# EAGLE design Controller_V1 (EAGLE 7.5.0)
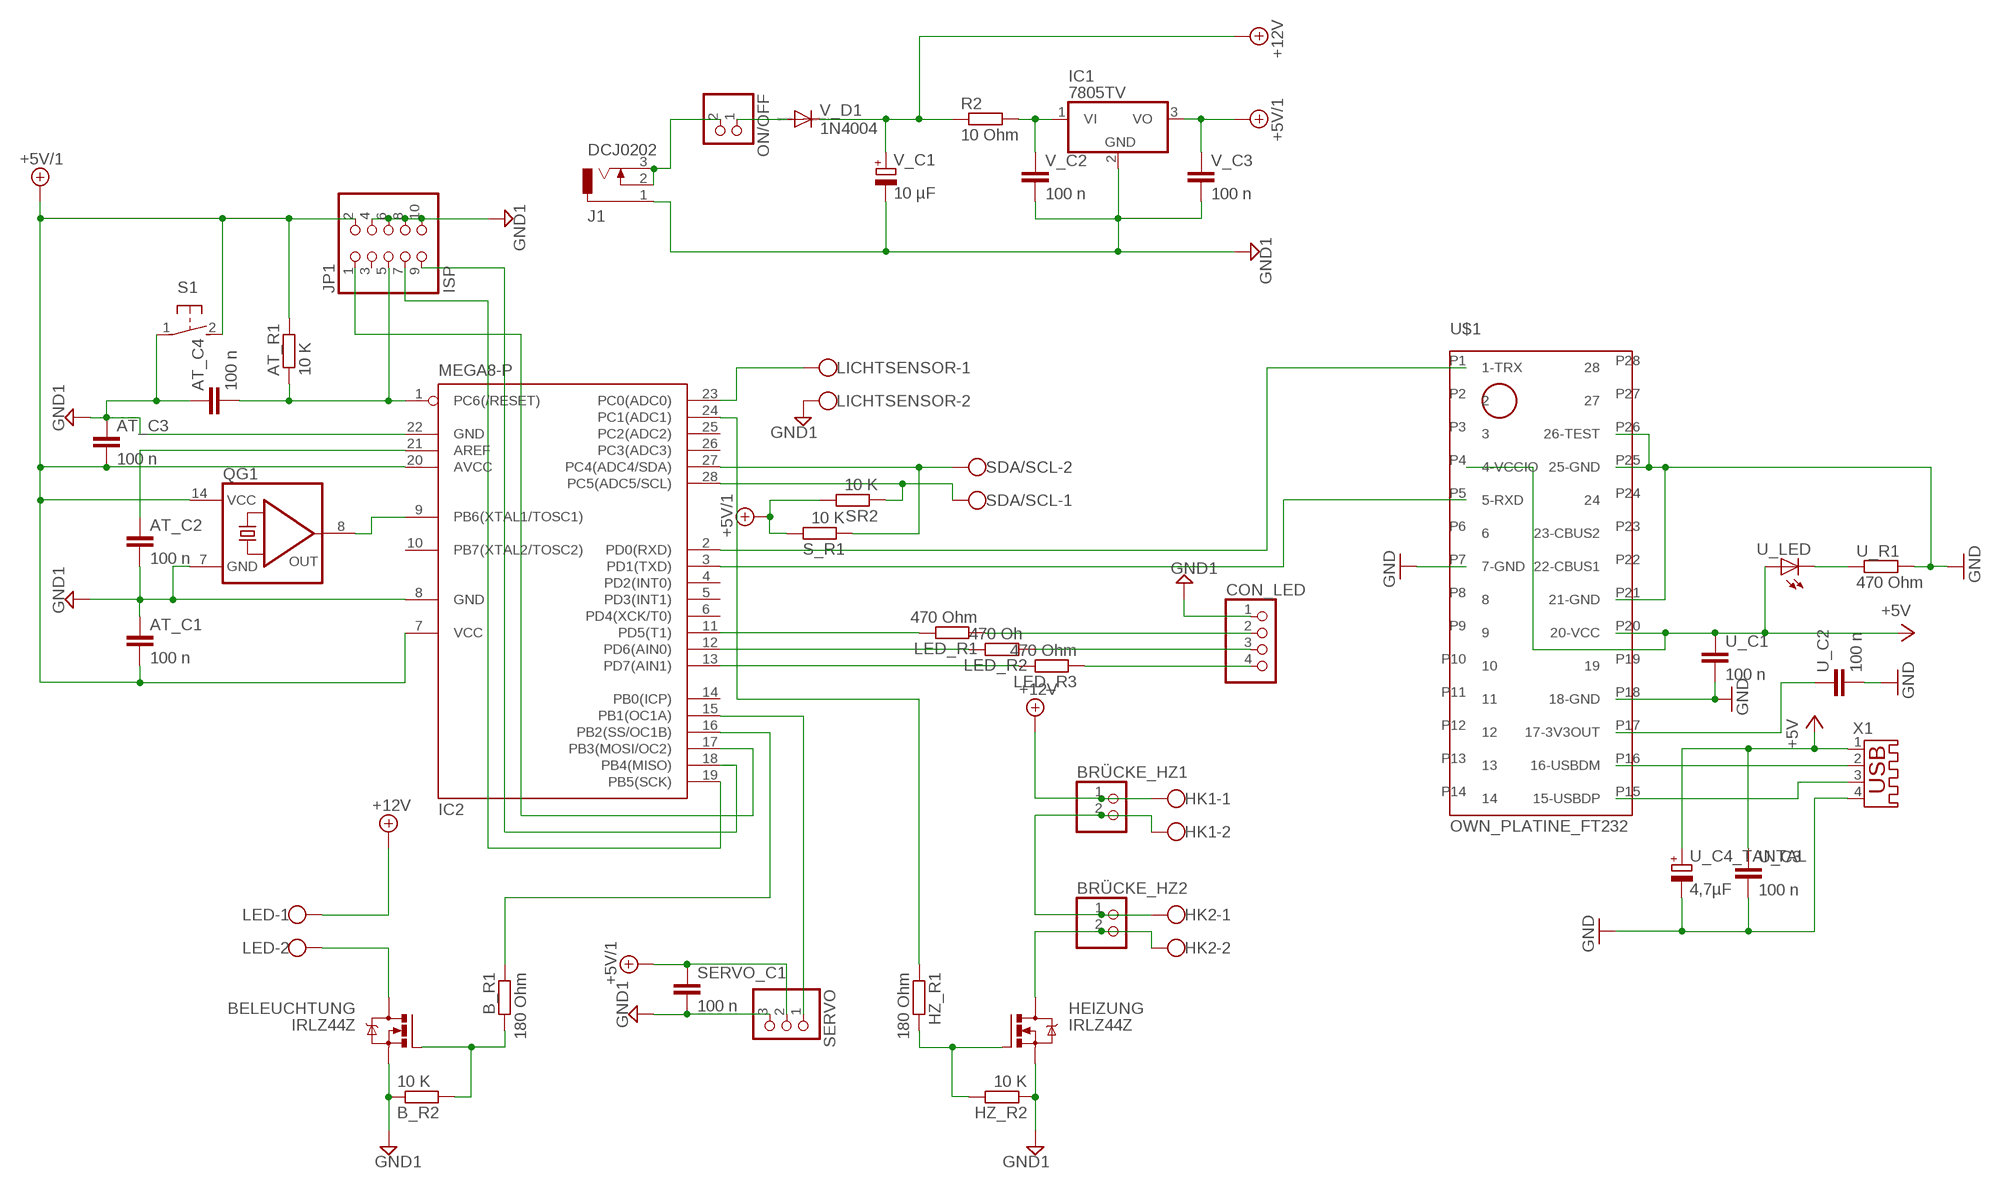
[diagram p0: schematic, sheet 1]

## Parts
AT_C1  100 n  C-EU025-025X050  [C025-025X050]
AT_C2  100 n  C-EU025-025X050  [C025-025X050]
AT_C3  100 n  C-EU025-025X050  [C025-025X050]
AT_C4  100 n  C-EU025-025X050  [C025-025X050]
AT_R1  10 K  R-EU_0204/7  [0204/7]
B_R1  180 Ohm  R-EU_0204/7  [0204/7]
B_R2  10 K  R-EU_0204/7  [0204/7]
BELEUCHTUNG  IRLZ44Z  [TO220BH]
BRÜCKE_HZ1  PINHD-1X2  [1X02]
BRÜCKE_HZ2  PINHD-1X2  [1X02]
CON_LED  PINHD-1X4  [1X04]
HEIZUNG  IRLZ44Z  [TO220BH]
HK1  W237-102  [W237-102]
HK2  W237-102  [W237-102]
HZ_R1  180 Ohm  R-EU_0204/7  [0204/7]
HZ_R2  10 K  R-EU_0204/7  [0204/7]
IC1  7805TV  [TO220V]
IC2  MEGA8-P  [DIL28-3]
J1  DCJ0202  [DCJ0202]
JP1  ISP  PINHD-2X5  [2X05]
LED  W237-102  [W237-102]
LED_R1  470 Ohm  R-EU_0204/7  [0204/7]
LED_R2  470 Oh  R-EU_0204/7  [0204/7]
LED_R3  470 Ohm  R-EU_0204/7  [0204/7]
LICHTSENSOR  W237-102  [W237-102]
ON/OFF  PINHD-1X2  [1X02]
QG1  QG5860  [DIL14S]
R2  10 Ohm  R-EU_0204/7  [0204/7]
S1  31-XX  [B3F-31XX]
S_R1  10 K  R-EU_0204/7  [0204/7]
SDA/SCL  W237-102  [W237-102]
SERVO  PINHD-1X3  [1X03]
SERVO_C1  100 n  C-EU025-025X050  [C025-025X050]
SR2  10 K  R-EU_0204/7  [0204/7]
U$1  OWN_PLATINE_FT232  [OWN_PLATINE_FT232]
U_C1  100 n  C-EU025-025X050  [C025-025X050]
U_C2  100 n  C-EU025-025X050  [C025-025X050]
U_C3  100 n  C-EU025-025X050  [C025-025X050]
U_C4_TANTAL  4,7µF  CPOL-EUE2,5-6E  [E2,5-6E]
U_LED  LED3MM  [LED3MM]
U_R1  470 Ohm  R-EU_0204/7  [0204/7]
V_C1  10 µF  CPOL-EUE2,5-6E  [E2,5-6E]
V_C2  100 n  C-EU025-025X050  [C025-025X050]
V_C3  100 n  C-EU025-025X050  [C025-025X050]
V_D1  1N4004  [DO41-10]
X1  USB-A003  [USB-A003]

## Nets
+5V: U$1.P4(4-VCCIO) U$1.P20(20-VCC) U_C1.1 U_C3.1 U_C4_TANTAL.+ U_LED.A X1.1
+5V/1: AT_C1.2 AT_C3.2 AT_R1.2 IC1.3(VO) IC2.7(VCC) IC2.20(AVCC) JP1.2 QG1.14(VCC) S1.2(S) S_R1.2 SERVO.2 SERVO_C1.1 SR2.2 V_C3.1
+12V: BRÜCKE_HZ1.1 HK1.1 LED.1 R2.1 V_C1.+ V_D1.C
AT_C1: IC2.2(PD0(RXD)) U$1.P1(1-TRX)
BELEUCHTUNG: BELEUCHTUNG.D LED.2
GND: U$1.P7(7-GND) U$1.P18(18-GND) U$1.P21(21-GND) U$1.P25(25-GND) U$1.P26(26-TEST) U_C1.2 U_C2.2 U_C3.2 U_C4_TANTAL.- U_R1.2 X1.4
GND1: AT_C1.1 AT_C2.2 AT_C3.1 AT_C4.1 B_R2.1 BELEUCHTUNG.S CON_LED.1 HEIZUNG.S HZ_R2.1 IC1.2(GND) IC2.8(GND) IC2.22(GND) J1.1 JP1.4 JP1.6 JP1.8 JP1.10 LICHTSENSOR.2 QG1.7(GND) S1.1(P) SERVO.3 SERVO_C1.2 V_C1.- V_C2.2 V_C3.2
N$1: U$1.P15(15-USBDP) X1.3
N$2: U$1.P17(17-3V3OUT) U_C2.1
N$3: U$1.P16(16-USBDM) X1.2
N$4: U_LED.K(C) U_R1.1
N$5: IC2.9(PB6(XTAL1/TOSC1)) QG1.8(OUT)
N$6: AT_C4.2 AT_R1.1 IC2.1(PC6(/RESET)) JP1.5
N$7: IC1.1(VI) R2.2 V_C2.1
N$9: AT_C2.1 IC2.21(AREF)
N$10: IC2.18(PB4(MISO)) JP1.9
N$11: J1.2 J1.3 ON/OFF.2
N$12: IC2.17(PB3(MOSI/OC2)) JP1.1
N$13: IC2.19(PB5(SCK)) JP1.7
N$14: IC2.3(PD1(TXD)) U$1.P5(5-RXD)
N$15: IC2.27(PC4(ADC4/SDA)) S_R1.1 SDA/SCL.2
N$16: IC2.28(PC5(ADC5/SCL)) SDA/SCL.1 SR2.1
N$17: IC2.15(PB1(OC1A)) SERVO.1
N$18: BRÜCKE_HZ1.2 BRÜCKE_HZ2.1 HK1.2 HK2.1
N$19: B_R1.2 B_R2.2 BELEUCHTUNG.G
N$20: HEIZUNG.G HZ_R1.2 HZ_R2.2
N$21: B_R1.1 IC2.16(PB2(SS/OC1B))
N$22: IC2.23(PC0(ADC0)) LICHTSENSOR.1
N$23: HZ_R1.1 IC2.24(PC1(ADC1))
N$24: BRÜCKE_HZ2.2 HEIZUNG.D HK2.2
N$25: IC2.13(PD7(AIN1)) LED_R3.2
N$26: CON_LED.2 LED_R1.1
N$27: CON_LED.3 LED_R2.1
N$28: CON_LED.4 LED_R3.1
N$29: IC2.11(PD5(T1)) LED_R1.2
N$30: IC2.12(PD6(AIN0)) LED_R2.2
ON/OFF: ON/OFF.1 V_D1.A
Unconnected: IC2.4(PD2(INT0)) IC2.5(PD3(INT1)) IC2.6(PD4(XCK/T0)) IC2.10(PB7(XTAL2/TOSC2)) IC2.14(PB0(ICP)) IC2.25(PC2(ADC2)) IC2.26(PC3(ADC3)) JP1.3 U$1.P2 U$1.P3 U$1.P6 U$1.P8 U$1.P9 U$1.P10 U$1.P11 U$1.P12 U$1.P13 U$1.P14 U$1.P19 U$1.P22(22-CBUS1) U$1.P23(23-CBUS2) U$1.P24 U$1.P27 U$1.P28

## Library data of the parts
AT_C1-AT_C4 SERVO_C1 U_C1-U_C3 V_C2 V_C3 = rcl:C-EU: CAPACITOR, European symbol
AT_R1 B_R1 B_R2 HZ_R1 HZ_R2 LED_R1-LED_R3 R2 S_R1 SR2 U_R1 = rcl:R-EU_: RESISTOR, European symbol
BELEUCHTUNG HEIZUNG = transistor-power:IRLZ44Z: N-Channel HEXFET® Power MOSFET Logic Level AUTOMOTIVE MOSFET Source: http://www.irf.com/product-info/datasheets/data/irlz44zpbf.pdf
BRÜCKE_HZ1 BRÜCKE_HZ2 ON/OFF = pinhead:PINHD-1X2: PIN HEADER
CON_LED = pinhead:PINHD-1X4: PIN HEADER
HK1 HK2 LED LICHTSENSOR SDA/SCL = con-wago-500:W237-102: WAGO SCREW CLAMP; MPN: 237-102; OC_FARNELL: unknown; OC_NEWARK: 70K9898
IC1 = linear:78*: Positive VOLTAGE REGULATOR Source: http://cache.national.com/ds/LM/LM78L05.pdf http://www.fairchildsemi.com/ds/LM/LM7805.pdf
IC2 = atmel:MEGA8-P: MICROCONTROLLER 8 Kbytes FLASH, 1 kbytes SRAM, 512 bytes EEPROM, USART, 4-channel 10 bit ADC, 2-channel 8 bit ADC Pin compatible with Atmega48, ATMega88, ATMega168 Source: avr.lbr; OC_FARNELL: unknown; OC_NEWARK: unknown
J1 = con-jack:DCJ0202: DC POWER JACK Source: DCJ0202.pdf; OC_FARNELL: unknown; OC_NEWARK: unknown
JP1 = pinhead:PINHD-2X5: PIN HEADER
QG1 = crystal:QG5860: CRYSTAL RESONATOR; OC_FARNELL: unknown; OC_NEWARK: unknown
S1 = switch-omron:31-XX: OMRON SWITCH; MPN: B3F-3100; OC_FARNELL: 959704; OC_NEWARK: 36M3582
SERVO = pinhead:PINHD-1X3: PIN HEADER
U$1 = own_USB_FT232_Platine:OWN_PLATINE_FT232
U_C4_TANTAL V_C1 = rcl:CPOL-EU: POLARIZED CAPACITOR, European symbol
U_LED = led:LED: LED
V_D1 = diode:1N4004: DIODE
X1 = con-yamaichi:USB-A003: USB connector; OC_FARNELL: unknown; OC_NEWARK: unknown

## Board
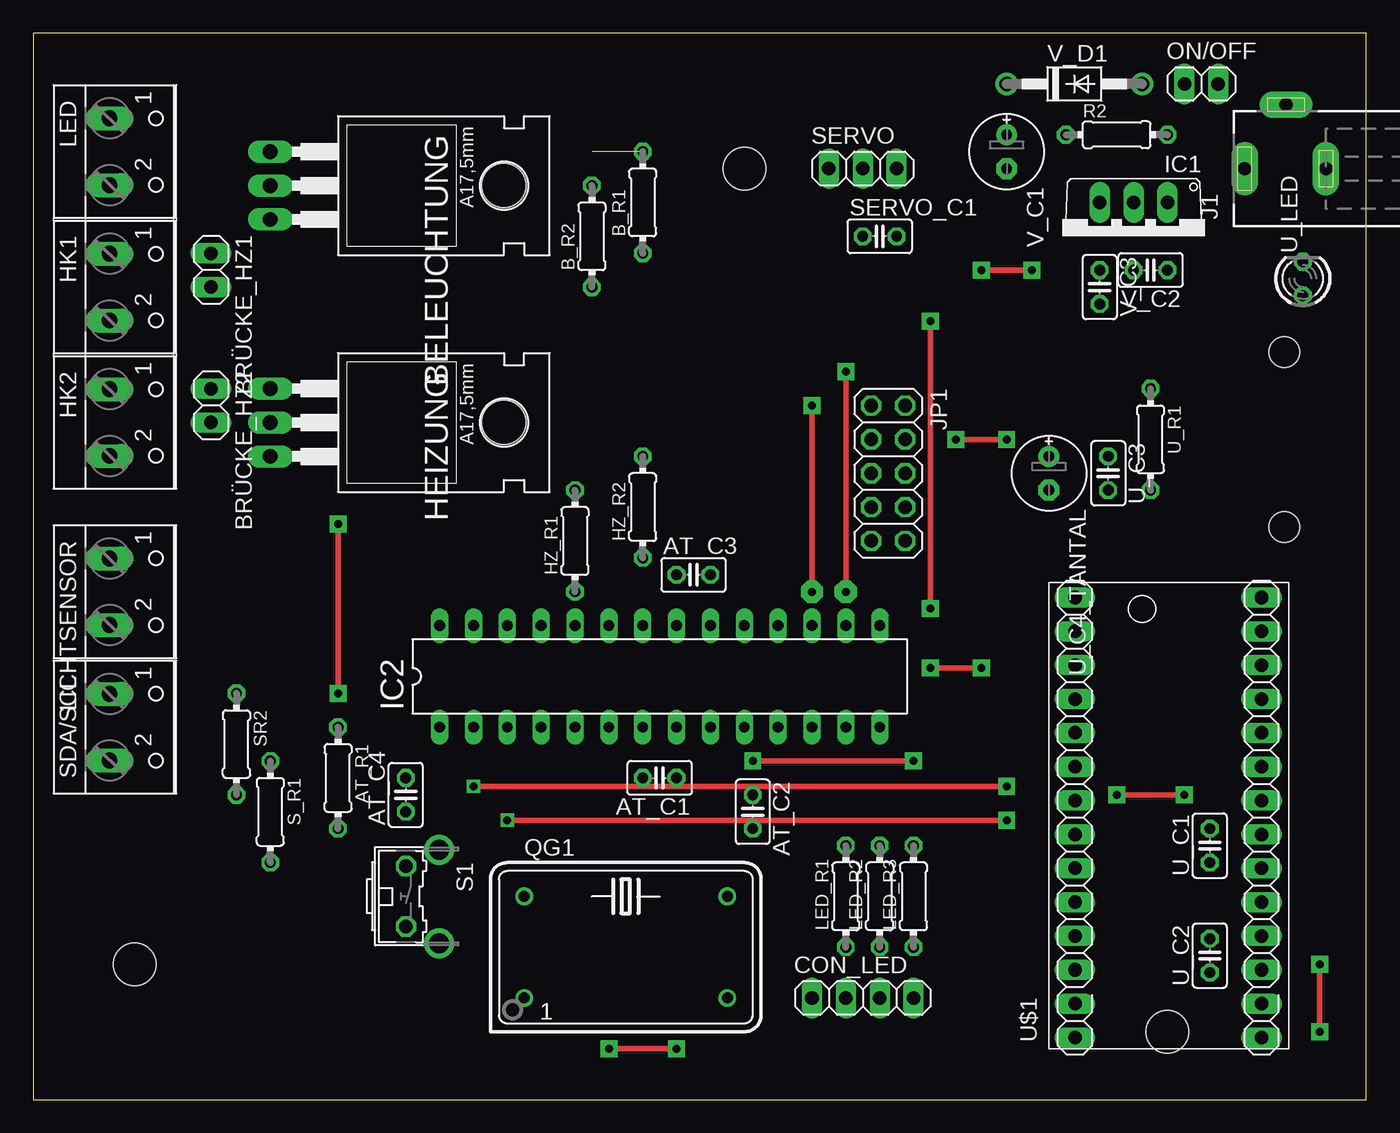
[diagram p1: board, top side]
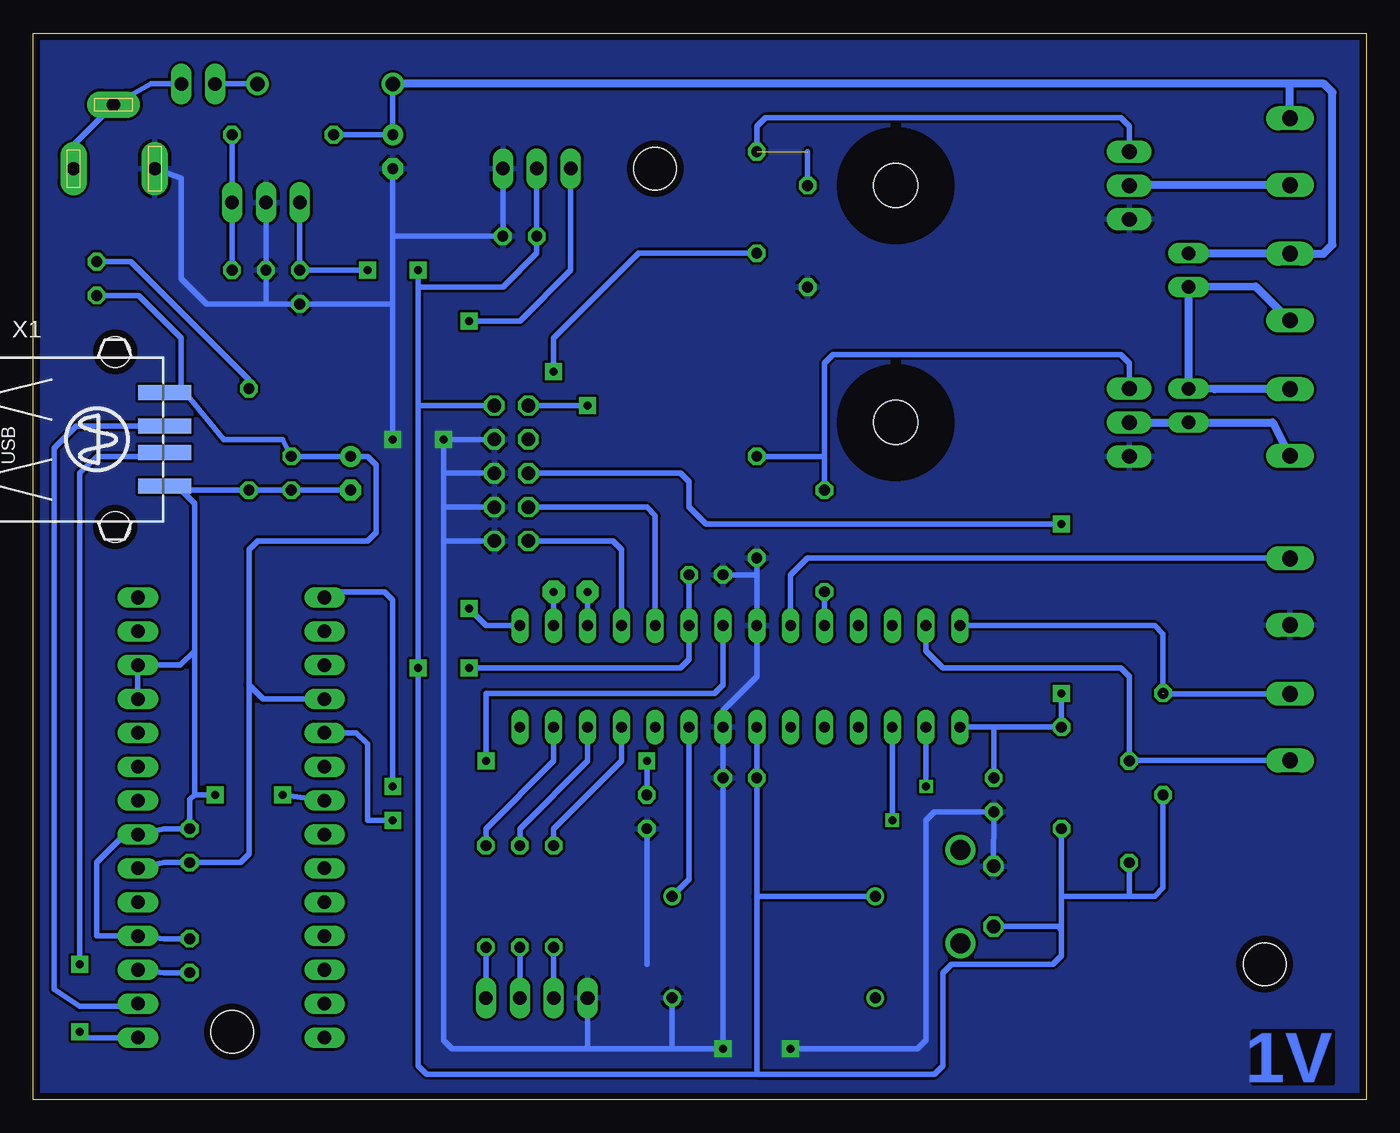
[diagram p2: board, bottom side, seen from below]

Size 100 x 80 mm. Coordinates in mm from the lower left corner, seen from the top.
Outline: 0,0 100,0 100,80 0,80 0,0
Copper layers (1*16): Top 0.035mm / dielectric 5mm / Bottom 0.035mm
Design rules "Controller_V1": minimum track width 10mil, minimum drill 10mil, track to track 0.205mm, track to pad 0.205mm, pad to pad 0.205mm, via to via 0.205mm, smd to smd 8mil, copper to edge 20mil, drill to drill 8mil, minimum pad ring 10mil, minimum via ring 8mil, stop-mask expansion 4mil, vias tented up to drill 0mil, thermal gap 10mil
Holes 3.2 mm at 7.62,10.16 53.34,69.85 85.09,5.08

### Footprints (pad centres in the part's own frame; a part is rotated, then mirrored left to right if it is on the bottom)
C025-025X050 = drill 0.813 octagon: 1 -1.27,0; 2 1.27,0
0204/7 = drill 0.813 octagon: 1 -3.81,0; 2 3.81,0
TO220BH = drill 1.118 long: D 0,-6.35; G -2.54,-6.35; S 2.54,-6.35 | hole 3.302: 0,11.176
1X02 = drill 1.016 long: 1 -1.27,0; 2 1.27,0
1X04 = drill 1.016 long: 1 -3.81,0; 2 -1.27,0; 3 1.27,0; 4 3.81,0
W237-102 = drill 1.194 long: 1 -2.5,-1.27; 2 2.5,-1.27
TO220V = drill 1.016 long: 1 -2.54,-2.54; 2 0,-2.54; 3 2.54,-2.54
DIL28-3 = drill 0.813 long: 1 -16.51,-3.81; 2 -13.97,-3.81; 3 -11.43,-3.81; 4 -8.89,-3.81; 5 -6.35,-3.81; 6 -3.81,-3.81; 7 -1.27,-3.81; 8 1.27,-3.81; 9 3.81,-3.81; 10 6.35,-3.81; 11 8.89,-3.81; 12 11.43,-3.81; 13 13.97,-3.81; 14 16.51,-3.81; 15 16.51,3.81; 16 13.97,3.81; 17 11.43,3.81; 18 8.89,3.81; 19 6.35,3.81; 20 3.81,3.81; 21 1.27,3.81; 22 -1.27,3.81; 23 -3.81,3.81; 24 -6.35,3.81; 25 -8.89,3.81; 26 -11.43,3.81; 27 -13.97,3.81; 28 -16.51,3.81
DCJ0202 = drill 1 pad 2 long: 1 0,3.1; 2 4.8,0; 3 0,-3
2X05 = drill 1.016 octagon: 1 -5.08,-1.27; 2 -5.08,1.27; 3 -2.54,-1.27; 4 -2.54,1.27; 5 0,-1.27; 6 0,1.27; 7 2.54,-1.27; 8 2.54,1.27; 9 5.08,-1.27; 10 5.08,1.27
DIL14S = drill 0.813: 1 -7.62,-3.81; 7 7.62,-3.81; 8 7.62,3.81; 14 -7.62,3.81
B3F-31XX = drill 1.016 octagon: 1 -2.261,-1.245; 2 2.261,-1.245 | drill 1.499 pad 2.159: 3 -3.505,1.245; 4 3.505,1.245
1X03 = drill 1.016 long: 1 -2.54,0; 2 0,0; 3 2.54,0
OWN_PLATINE_FT232 = drill 1.016 long: P1 1.95,33.86; P2 1.95,31.32; P3 1.95,28.78; P4 1.95,26.24; P5 1.95,23.7; P6 1.95,21.16; P7 1.95,18.62; P8 1.95,16.08; P9 1.95,13.54; P10 1.95,11; P11 1.95,8.46; P12 1.95,5.92; P13 1.95,3.38; P14 1.95,0.84; P15 15.95,0.84; P16 15.95,3.38; P17 15.95,5.92; P18 15.95,8.46; P19 15.95,11; P20 15.95,13.54; P21 15.95,16.08; P22 15.95,18.62; P23 15.95,21.16; P24 15.95,23.7; P25 15.95,26.24; P26 15.95,28.78; P27 15.95,31.32; P28 15.95,33.86
E2,5-6E = drill 0.813 pad 1.575: + -1.27,0 | drill 0.813 pad 1.575 octagon: - 1.27,0
LED3MM = drill 0.813 octagon: A -1.27,0; K 1.27,0
DO41-10 = drill 1.118: A 5.08,0; C -5.08,0
USB-A003 = smd 1.12 x 4: 1 -3.5,14; 2 -1,14; 3 1,14; 4 3.5,14 | hole 2.3: -6.57,10.28; 6.57,10.28

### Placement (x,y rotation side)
AT_C1  46.99,24.13 180 top
AT_C2  53.98,21.59 270 top
AT_C3  49.53,39.37 0 top
AT_C4  27.94,22.86 90 top
AT_R1  22.86,24.13 270 top
B_R1  45.72,67.31 90 top
B_R2  41.91,64.77 90 top
BELEUCHTUNG  24.13,68.58 270 top
BRÜCKE_HZ1  13.34,62.23 270 top
BRÜCKE_HZ2  13.34,52.07 270 top
CON_LED  62.23,7.62 0 top
HEIZUNG  24.13,50.8 270 top
HK1  6.99,60.96 270 top
HK2  6.99,50.8 270 top
HZ_R1  40.64,41.91 90 top
HZ_R2  45.72,44.45 90 top
IC1  82.55,64.77 180 top
IC2  46.99,31.75 0 top
J1  93.98,69.85 90 top
JP1  64.14,46.99 270 top
LED  6.99,71.12 270 top
LED_R1  60.96,15.24 90 top
LED_R2  63.5,15.24 90 top
LED_R3  66.04,15.24 90 top
LICHTSENSOR  6.99,38.1 270 top
ON/OFF  87.63,76.2 0 top
QG1  44.45,11.43 0 top
R2  81.28,72.39 0 top
S1  29.21,15.24 270 top
S_R1  17.78,21.59 270 top
SDA/SCL  6.99,27.94 270 top
SERVO  62.23,69.85 0 top
SERVO_C1  63.5,64.77 0 top
SR2  15.24,26.67 270 top
U$1  76.2,3.81 0 top
U_C1  88.27,19.05 90 top
U_C2  88.27,10.79 90 top
U_C3  80.64,46.99 270 top
U_C4_TANTAL  76.2,46.99 270 top
U_LED  95.25,61.59 90 top
U_R1  83.82,49.53 270 top
V_C1  73.03,71.12 270 top
V_C2  83.82,62.23 180 top
V_C3  80.01,60.96 270 top
V_D1  78.11,76.2 0 top
X1  104.14,49.53 270 bottom

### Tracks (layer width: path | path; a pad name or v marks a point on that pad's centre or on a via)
+5V
  Bottom 0.406: U_C3.1 81.28,49.53 85.72,49.53 88.59,53.03 X1.1 88.9,53.06 88.9,57.15 92.08,60.33 U_LED.A | U_C4_TANTAL.+ U_C3.1 | U_C3.1 74.93,48.26 74.3,47.62 74.3,42.55 74.93,41.91 83.19,41.91 83.82,41.27 83.82,31.11 | 83.82,31.11 83.82,18.41 84.45,17.78 U_C1.1 90.17,17.78 U$1.P20 | U$1.P4 82.75,30.05 83.82,31.11
+5V/1  (via drill 0.6, 0.6 pad 1.27)
  Top 0.406: v74.93,62.23 v71.12,62.23 | v67.31,32.38 v71.12,32.38
  Bottom 0.406: IC1.3 V_C3.1 v74.93,62.23 | IC2.7 AT_C1.2 45.72,15.24 | AT_C3.2 IC2.20 50.8,33.02 51.44,32.38 v67.31,32.38 | 71.12,52.07 v71.12,32.38 71.12,2.54 70.48,1.91 45.72,1.91 | 71.12,52.07 71.12,60.96 | 71.12,60.96 v71.12,62.23 | AT_R1.2 22.86,15.24 | 22.86,15.24 22.86,12.7 | JP1.2 71.12,52.07 | S1.2 23.14,12.98 22.86,12.7 | 45.72,15.24 45.72,1.91 | QG1.14 45.72,15.24 | SERVO.2 SERVO_C1.1 62.23,63.5 64.77,60.96 71.12,60.96 | SR2.2 15.24,15.88 15.88,15.24 17.78,15.24 | 17.78,15.24 22.86,15.24 | 45.72,1.91 32.38,1.91 31.75,2.54 31.75,9.53 31.11,10.16 23.5,10.16 22.86,10.79 22.86,12.7 | S_R1.2 17.78,15.24
+12V
  Bottom 0.406: V_D1.C V_C1.+ R2.1 | 13.93,63.46 BRÜCKE_HZ1.1
  Bottom 0.61: 13.93,63.46 HK1.1 3.21,63.46 2.54,64.14 2.54,75.56 3.17,76.2 5.71,76.2 | 5.71,76.2 V_D1.C | LED.1 5.71,76.2
AT_C1  (via drill 0.6, 0.6 pad 1.27)
  Top 0.406: v73.03,23.5 v33.02,23.5
  Bottom 0.406: U$1.P1 77.72,38.1 73.66,38.1 73.03,37.47 v73.03,23.5 | v33.02,23.5 IC2.2
BELEUCHTUNG
  Bottom 0.406: 19.01,68.62 BELEUCHTUNG.D
  Bottom 0.61: LED.2 19.01,68.62
GND  (via drill 0.6, 0.6 pad 1.27)
  Top 0.406: v81.28,22.86 v86.36,22.86
  Bottom 0.406: U_C4_TANTAL.- U_C3.2 U_R1.2 88.9,45.72 | X1.4 89.21,46.03 88.9,45.72 | U$1.P7 78.31,22.43 v81.28,22.86 | v86.36,22.86 87.91,22.86 | 87.91,22.86 87.91,33.66 | 87.91,33.66 87.91,44.73 88.9,45.72 | 87.91,33.66 88.97,32.59 U$1.P26 U$1.P25 | U_C2.2 90.17,12.06 U$1.P18 95.25,12.27 95.25,17.78 93.14,19.89 U$1.P21 90.17,20.32 U_C1.2 88.27,22.5 87.91,22.86
GND1  (via drill 0.6, 0.6 pad 1.27)
  Top 0.406: v43.18,3.81 v48.26,3.81 | v73.03,49.53 v69.22,49.53
  Bottom 0.406: J1.1 88.9,69.14 88.9,61.59 87,59.69 82.55,59.69 | 73.03,64.77 V_C1.- | JP1.4 v69.22,49.53 69.22,46.99 | 69.22,46.99 69.22,44.45 | 69.22,44.45 69.22,41.91 | JP1.6 69.22,46.99 | JP1.8 69.22,44.45 | JP1.10 69.22,41.91 | 69.22,41.91 69.22,4.45 68.58,3.81 58.42,3.81 | AT_C2.2 53.98,10.16 | CON_LED.1 58.42,3.81 | 58.42,3.81 52.07,3.81 | 52.07,3.81 v48.26,3.81 AT_C1.1 IC2.8 48.26,29.21 45.72,31.75 IC2.22 45.72,39.37 | QG1.7 52.07,3.81 | v43.18,3.81 33.66,3.81 33.02,4.45 33.02,20.95 32.38,21.59 AT_C4.1 S1.1 | 73.03,64.77 73.03,59.69 | 73.03,59.69 v73.03,49.53 | SERVO.3 SERVO_C1.2 73.03,64.77 | 73.03,59.69 V_C3.2 82.55,59.69 | IC1.2 V_C2.2 82.55,59.69 | HZ_R2.1 45.72,39.37 | AT_C3.1 45.72,39.37
  pour Bottom (isolate 0.203, rank 3): 0,80.01 100.33,80.01 100.33,0 0,0
N$1  (via drill 0.6, 0.6 pad 1.27)
  Top 0.406: v96.52,5.08 v96.52,10.16
  Bottom 0.406: U$1.P15 96.09,4.65 v96.52,5.08 | v96.52,10.16 96.52,46.99 95.25,48.26 89.14,48.26 X1.3
N$2
  Bottom 0.406: U_C2.1 90.17,9.53 U$1.P17
N$3
  Bottom 0.406: X1.2 96.79,50.53 98.42,48.9 98.42,8.26 96.52,6.99 92.58,6.99 U$1.P16
N$4
  Bottom 0.406: U_LED.K 92.71,62.87 83.82,53.98 U_R1.1
N$5
  Bottom 0.406: QG1.8 50.8,16.51 IC2.9
N$6  (via drill 0.6 pad 1.27)
  Top 0.406: v22.86,30.48 v22.86,43.18
  Bottom 0.406: 27.94,27.94 IC2.1 AT_R1.1 | 27.94,27.94 AT_R1.1 | AT_C4.2 27.94,27.94 | AT_R1.1 v22.86,30.48 | v22.86,43.18 49.53,43.18 50.8,44.45 50.8,46.35 51.44,46.99 JP1.5
N$7
  Bottom 0.406: V_C2.1 IC1.1 R2.2
N$9  (via drill 0.6, 0.6 pad 1.27)
  Top 0.406: v53.98,25.4 v66.04,25.4
  Bottom 0.406: AT_C2.1 v53.98,25.4 | v66.04,25.4 66.04,30.48 48.9,30.48 48.26,31.11 IC2.21
N$10
  Bottom 0.406: IC2.18 55.88,41.27 56.52,41.91 JP1.9
N$11
  Bottom 0.406: J1.3 96.98,71.65 J1.2 91.16,76.2 ON/OFF.2
N$12  (via drill 0.6, 0.6 pad 1.27, 0.6 pad 1.68)
  Top 0.406: v58.42,38.1 v58.42,52.07
  Bottom 0.406: IC2.17 v58.42,38.1 | v58.42,52.07 JP1.1
N$13
  Bottom 0.406: IC2.19 53.34,43.81 53.98,44.45 JP1.7
N$14  (via drill 0.6)
  Top 0.406: v73.03,20.95 v35.56,20.95
  Bottom 0.406: v35.56,20.95 IC2.3 | U$1.P5 75.77,27.51 74.93,26.67 74.93,20.95 v73.03,20.95
N$15
  Bottom 0.406: SDA/SCL.2 17.74,25.44 S_R1.1 17.78,31.75 18.41,32.38 31.75,32.38 33.02,33.66 IC2.27
N$16  (1 unrouted)
  Bottom 0.406: SDA/SCL.1 15.2,30.44 | SR2.1 15.24,34.92 15.88,35.56 IC2.28
N$17  (via drill 0.6, 0.6 pad 1.27)
  Top 0.406: v67.31,58.42 v67.31,36.83
  Bottom 0.406: SERVO.1 59.69,62.23 63.5,58.42 v67.31,58.42 | v67.31,36.83 66.04,35.56 IC2.15
N$18
  Bottom 0.61: HK1.2 8.29,61 BRÜCKE_HZ1.2 BRÜCKE_HZ2.1 11.39,53.3 HK2.1
N$19  (1 unrouted)
  Bottom 0.406: B_R2.2 41.91,71.12 | BELEUCHTUNG.G 17.78,73.03 18.41,73.66 45.09,73.66 45.72,73.03 B_R1.2
N$20
  Bottom 0.406: 40.64,48.26 40.64,55.24 40.01,55.88 18.41,55.88 17.78,55.24 HEIZUNG.G | 40.64,48.26 HZ_R1.2 | HZ_R2.2 40.64,48.26
N$21  (via drill 0.6, 0.6 pad 1.27, 0.6 pad 1.68)
  Top 0.406: v60.96,38.1 v60.96,54.61
  Bottom 0.406: IC2.16 v60.96,38.1 | v60.96,54.61 60.96,57.15 54.61,63.5 B_R1.1
N$22
  Bottom 0.406: IC2.23 43.18,39.37 41.91,40.64 6.35,40.64 6.31,40.6 LICHTSENSOR.1
N$23
  Bottom 0.406: HZ_R1.1 IC2.24
N$24
  Bottom 0.61: HK2.2 7.03,50.8 BRÜCKE_HZ2.2 HEIZUNG.D
N$25
  Bottom 0.406: IC2.13 60.96,25.4 66.04,20.32 LED_R3.2
N$26
  Bottom 0.406: LED_R1.1 CON_LED.2
N$27
  Bottom 0.406: LED_R2.1 CON_LED.3
N$28
  Bottom 0.406: LED_R3.1 CON_LED.4
N$29
  Bottom 0.406: IC2.11 55.88,25.4 60.96,20.32 LED_R1.2
N$30
  Bottom 0.406: IC2.12 58.42,25.4 63.5,20.32 LED_R2.2
N$31  (via drill 0.6 pad 1.27)
  other vias: 73.03,20.95
ON/OFF
  Bottom 0.406: ON/OFF.1 V_D1.A

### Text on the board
Bottom: 1V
